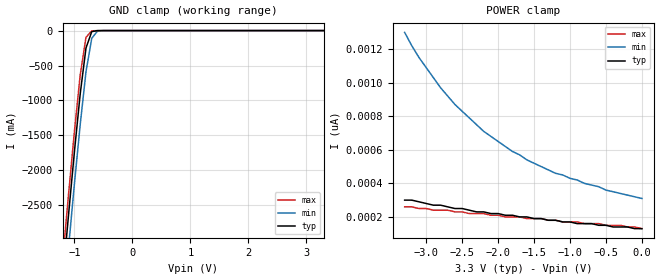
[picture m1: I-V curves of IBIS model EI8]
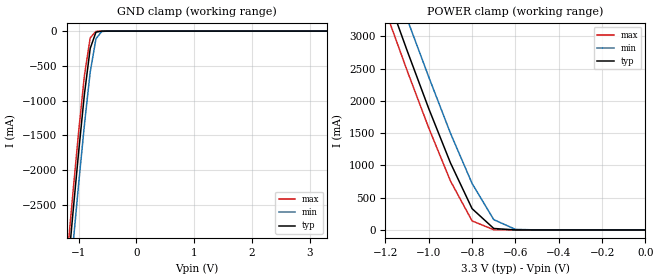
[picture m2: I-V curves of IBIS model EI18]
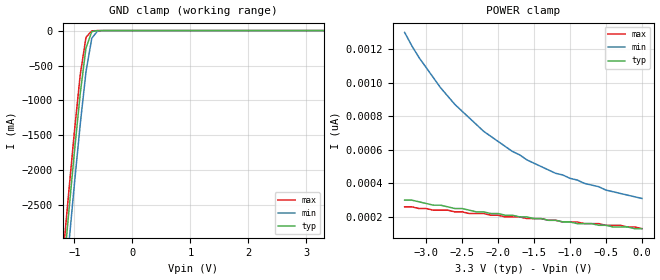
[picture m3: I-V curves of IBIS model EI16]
|   * 9fgp204b.ibs * IBIS 2.1 Model file
| Rev History
| Rev No.   Description
| 1.0   Initial release with Updated Parasitic Parameters April 7, 2010
| 1.1   Corrected 0 ohm Rref values September 8, 2010
[IBIS Ver]   2.1
[Comment char]  |_char
[File name]   9fgp204b.ibs
[Date]   September 8, 2010
[File Rev]   1.1
[Source]   Originated at Integrated Circuit Systems, Inc.
[Disclaimer] (C) Copyright Integrated Circuit Systems, Inc. 2004
   All rights reserved
ICS hereby grants the user of this IBIS model a non-exclusive,
nontransferable license to use this IBIS model under the following terms.
Before using this IBIS model, the user should read this license.
If the user does not accept these terms,  the IBIS model should be
returned to ICS within 30 days.
   The user is granted this license only to use the IBIS model and
is not granted rights to sell, load, rent, lease or license the IBIS
model in whole or in part, or in modified form to anyone other than
user. User may modify the IBIS model to suit its specific
applications but rights to derivative works and such modifications
shall belong to ICS.
   This IBIS model is provided on an "AS IS" basis and ICS makes
absolutely no warranty with respect to the information contained
herein. ICS DISCLAIMS AND CUSTOMER WAIVES ALL WARRANTIES, EXPRESS
OR IMPLIED, INCLUDING WARRANTIES OF MERCHANTABILITY OR FITNESS FOR
A PARTICULAR PURPOSE. The entire risk as to quality and performance
is with the Customer. ACCORDINGLY, IN NO EVENT SHALL THE COMPANY BE
LIABLE FOR ANY DAMAGES, WHETHER IN CONTRACT OR TORT,INCLUDING ANY
LOST PROFITS OR OTHER INCIDENTAL, CONSEQUENTIAL, EXEMPLARY, OR
model provided in this package. Further, ICS reserves the right to
make changes without notice to any product herein to improve
reliability, function, or design. ICS does not convey any license
under patent rights or any other intellectual property rights,
including those of third parties.
   ICS is not obligated to provide maintenance or support
for the licensed IBIS model.
There are 2 components in this IBIS file:
1. ICS9FGP204B_1X
   RMII : 1X
   33.33MHz : 1X
   25MHz : 1X
   32.768MHz  : 1X
2. ICS9FGP204B_2X
   RMII : 2X
   33.33MHz : 2X
   25MHz : 2X
   32.768MHz  : 2X
|   COMPONENT: ICS9FGP204B_1X
[Component]   ICS9FGP204B_1X
[Manufacturer]  ICS
[Package]
| variable   typ   min   max
R_pkg   81.1m   62.2m   100.0m
L_pkg   6.7nH   4.9nH   8.5nH
C_pkg   0.53pF  0.21pF  0.85pF
[Pin]   signal_name   model_name   R_pin   L_pin   C_pin
  1   GND   GND
  2   VDD96   POWER
  3   DOT96SST   EH6
  4   DOT96SSC   EH6
  5   OE_96   EI18
  6   OE_CPU   EI18
  7   CPUCLKT0   EH6
  8   CPUCLKC0   EH6
  9   VDDCPU   POWER
 10   GNDCPU   GND
 11   IREF   NC
 12   VDD32K   POWER
 13   32.768KHz   EO30
 14   GND32K   GND
 15   VDDREF   POWER
 16   25MHz_0   EO30
 17   25MHz_1   EO30
 18   GNDREF   GND
 19   X1_25   EIX
 20   X2_25   EIX
 21   GND33   GND
 22   33.33MHz/SMBADR   EIO34d
 23   VDD33   POWER
 24   RMII5   EO30
 25   RMII4   EO30
 26   VDDRMII   POWER
 27   GNDRMII   GND
 28   RMII3   EO30
 29   RMII2   EO30
 30   GNDRMII   GND
 31   VDDRMII   POWER
 32   RMII1   EO30
 33   RMII0   EO30
 34   VDDRGMII   POWER
 35   GNDRGMII   GND
 36   RGMII1   EO34
 37   RGMII0   EO34
 38   SCLK   EI8
 39   SDATA   EIOD1
 40   VTTPWR_GD/PD#   EI16
|* Either 3.3V or 2.5V
|** All model are simulated with typical corner process
[Diff Pin]   inv_pin   vdiff   tdelay_typ
3   4   NA   NA
7   8   NA   NA
|   COMPONENT: ICS9FGP204B_2X
[Component]   ICS9FGP204B_2X
[Manufacturer]  ICS
[Package]
| variable   typ   min   max
R_pkg   81.1m   62.2m   100.0m
L_pkg   6.7nH   4.9nH   8.5nH
C_pkg   0.53pF  0.21pF  0.85pF
[Pin]   signal_name   model_name   R_pin   L_pin   C_pin
  1   GND   GND
  2   VDD96   POWER
  3   DOT96SST   EH6
  4   DOT96SSC   EH6
  5   OE_96   EI18
  6   OE_CPU   EI18
  7   CPUCLKT0   EH6
  8   CPUCLKC0   EH6
  9   VDDCPU   POWER
 10   GNDCPU   GND
 11   IREF   NC
 12   VDD32K   POWER
 13   32.768KHz   EO31
 14   GND32K   GND
 15   VDDREF   POWER
 16   25MHz_0   EO31
 17   25MHz_1   EO31
 18   GNDREF   GND
 19   X1_25   EIX
 20   X2_25   EIX
 21   GND33   GND
 22   33.33MHz/SMBADR   EIO35d
 23   VDD33   POWER
 24   RMII5   EO31
 25   RMII4   EO31
 26   VDDRMII   POWER
 27   GNDRMII   GND
 28   RMII3   EO31
 29   RMII2   EO31
 30   GNDRMII   GND
 31   VDDRMII   POWER
 32   RMII1   EO31
 33   RMII0   EO31
 34   VDDRGMII   POWER
 35   GNDRGMII   GND
 36   RGMII1   EO34
 37   RGMII0   EO34
 38   SCLK   EI8
 39   SDATA   EIOD1
 40   VTTPWR_GD/PD#   EI16
|* Either 3.3V or 2.5V
|** All model are simulated with typical corner process
[Diff Pin]   inv_pin   vdiff   tdelay_typ
3   4   NA   NA
7   8   NA   NA
| Models and submodels in the file (11): EI8 (Input), EI18 (Input), EI16 (Input), EIO34d (I/O), EIO35d (I/O), EIOD1 (I/O_open_drain), EIX (Input), EH6 (Open_source), EO30 (Output), EO31 (Output), EO34 (Output)
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|   Model EI8
[Model]   EI8
Model_type   Input
Polarity   Inverting
Vinl =   0.80V
Vinh =   2.00V
C_comp   3.40pF   2.85pF   3.95pF
[Temperature Range]   27.00   70.00   0.000
[Voltage Range]   3.30V   3.00V   3.70V
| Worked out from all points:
|   GND clamp passes 1 mA (typ) near -0.60 V on its own axis
[GND_clamp]
| voltage   I(typ)   I(min)   I(max)
-3.3V     -24.05A    -24.49A    -23.79A
-1.2V     -3.55A     -4.02A     -3.26A
-1.1V     -2.63A     -3.1A      -2.34A
-1V       -1.74A     -2.2A      -1.45A
-900mV    -910mA     -1.35A     -640mA
-800mV    -250mA     -590mA     -96.82mA
-700mV    -14.58mA   -110mA     -3.87mA
-600mV    -880uA     -5.84mA    -450uA
-500mV    -88.5uA    -350uA     -45.09uA
3.3V      130pA      340pA      120pA
[POWER_clamp]
| voltage   I(typ)   I(min)   I(max)
-3.3V     300pA      1.3nA      260pA
-3.1V     290pA      1.15nA     250pA
-2.9V     270pA      1.03nA     240pA
-2.8V     270pA      970pA      240pA
-2.6V     250pA      870pA      230pA
-2.2V     230pA      710pA      220pA
-1.8V     210pA      590pA      200pA
-1.2V     180pA      460pA      180pA
-900mV    160pA      420pA      170pA
-500mV    150pA      360pA      150pA
-300mV    140pA      340pA      150pA
0V        130pA      310pA      130pA
|   Model EI18
[Model]   EI18
Model_type   Input
Enable   Active-High
Vinl =   0.80V
Vinh =   2.00V
C_comp   3.40pF   2.85pF   3.95pF
[Temperature Range]   27.00   70.00   0.000
[Voltage Range]   3.30V   3.00V   3.70V
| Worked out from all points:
|   GND clamp passes 1 mA (typ) near -0.60 V on its own axis
|   POWER clamp passes 1 mA (typ) near -0.60 V on its own axis
[GND_clamp]
| voltage   I(typ)   I(min)   I(max)
-3.3V     -24.05A    -24.49A    -23.79A
-1.2V     -3.55A     -4.02A     -3.26A
-1.1V     -2.63A     -3.1A      -2.34A
-1V       -1.74A     -2.2A      -1.45A
-900mV    -910mA     -1.35A     -640mA
-800mV    -250mA     -590mA     -96.82mA
-700mV    -14.58mA   -110mA     -3.87mA
-600mV    -880uA     -5.82mA    -450uA
-500mV    -88.5uA    -350uA     -45.09uA
3.3V      130pA      470nA      90.8pA
[POWER_clamp]
| voltage   I(typ)   I(min)   I(max)
-3.3V     24.22A     24.68A     23.94A
-1.2V     3.71A      4.2A       3.4A
-1.1V     2.78A      3.27A      2.47A
-1V       1.88A      2.37A      1.58A
-900mV    1.04A      1.5A       760mA
-800mV    330mA      720mA      140mA
-700mV    23.1mA     160mA      3.86mA
-600mV    560uA      9.44mA     65.29uA
0V        130pA      310pA      130pA
|   Model EI16
[Model]   EI16
Model_type   Input
Polarity   Non-Inverting
Vinl =   0.80V
Vinh =   2.00V
C_comp   3.40pF   2.85pF   3.95pF
[Temperature Range]   27.00   70.00   0.000
[Voltage Range]   3.30V   3.00V   3.70V
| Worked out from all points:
|   GND clamp passes 1 mA (typ) near -0.60 V on its own axis
[GND_clamp]
| voltage   I(typ)   I(min)   I(max)
-3.3V     -24.05A    -24.48A    -23.79A
-1.2V     -3.55A     -4.02A     -3.26A
-1.1V     -2.63A     -3.1A      -2.34A
-1V       -1.74A     -2.2A      -1.45A
-900mV    -910mA     -1.35A     -640mA
-800mV    -250mA     -590mA     -96.82mA
-700mV    -14.58mA   -110mA     -3.87mA
-600mV    -880uA     -5.82mA    -450uA
-500mV    -88.5uA    -350uA     -45.09uA
3.3V      130pA      340pA      120pA
[POWER_clamp]
| voltage   I(typ)   I(min)   I(max)
-3.3V     300pA      1.3nA      260pA
-3.1V     290pA      1.15nA     250pA
-2.9V     270pA      1.03nA     240pA
-2.8V     270pA      970pA      240pA
-2.6V     250pA      870pA      230pA
-2.2V     230pA      710pA      220pA
-1.8V     210pA      590pA      200pA
-1.2V     180pA      460pA      180pA
-900mV    160pA      420pA      170pA
-500mV    150pA      360pA      150pA
-300mV    140pA      340pA      150pA
0V        130pA      310pA      130pA
